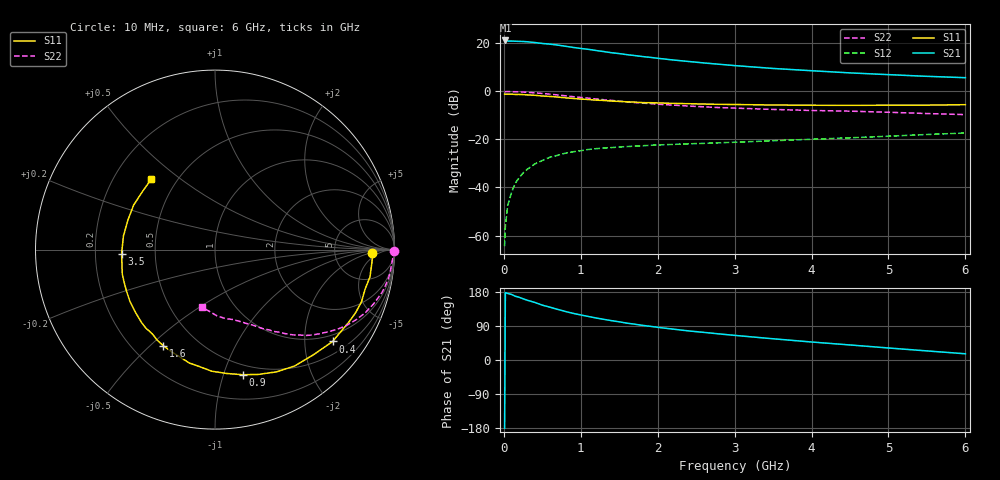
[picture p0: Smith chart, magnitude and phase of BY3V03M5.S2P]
! SIEMENS Small Signal Semiconductors
! BFY420
! Si NPN RF SIEGET Grounded Emitter Transistor in MICRO-X
! VCE = 3 V  IC = 3.5 mA
! Common Emitter S-Parameters:  October  1996
# GHz  S  MA  R  50
!  f  S11  S21  S12  S22
! GHz  MAG  ANG  MAG  ANG  MAG  ANG  MAG  ANG
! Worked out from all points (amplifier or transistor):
!   36 points, 10 MHz to 6 GHz, reference 50 ohm
!   highest |S21| = 21.2 dB at 20 MHz (marker M1)
!   |S21| within 3 dB of that: start of sweep to 924.5 MHz
!   unconditionally stable (mu >= 1): 3.483 GHz to end of sweep
!   at 250 MHz: K = 0.09, MSG = 27.4 dB, |S12| = -33.9 dB
!   at 1.4 GHz: K = 0.42, MSG = 19.7 dB, |S12| = -23.4 dB
!   at 6 GHz: K = 1.18, MAG = 9.0 dB, |S12| = -17.3 dB
!   S11 on the Smith chart (normalised r, x): 10 MHz: 15, -2; 400 MHz: 0.81, -2.69; 900 MHz: 0.41, -1.16; 1.6 GHz: 0.32, -0.55; 3.5 GHz: 0.32, -0.02; 6 GHz: 0.36, +0.39
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0.01  0.8764 -1.1  11.45 -180.0  0.0006 74.6  0.995 -0.4
0.02  0.8788 -2.2  11.51 177.9  0.0016 88.3  0.9864 -0.9
0.05  0.877 -5.0  11.19 175.6  0.0042 81.2  0.9926 -2.4
0.1  0.8767 -10.0  11.17 173.0  0.0079 83.1  0.9873 -4.9
0.15  0.8647 -14.7  11.09 168.2  0.0124 79.7  0.9842 -7.3
0.2  0.8665 -19.6  11.01 165.5  0.016 79.0  0.9794 -9.6
0.3  0.8474 -28.7  10.81 158.0  0.0236 74.3  0.9607 -14.4
0.4  0.8315 -38.0  10.44 152.1  0.0307 69.6  0.9347 -18.8
0.5  0.8031 -46.7  9.969 144.8  0.0364 65.0  0.9074 -22.9
0.6  0.7856 -55.6  9.645 139.3  0.0428 61.0  0.8765 -26.6
0.7  0.763 -63.2  9.223 133.6  0.0468 57.2  0.8441 -30.2
0.9  0.7137 -77.6  8.246 123.1  0.0554 51.0  0.7789 -36.0
1.1  0.6779 -91.5  7.512 114.8  0.0619 45.9  0.7221 -41.2
1.3  0.6479 -102.8  6.752 107.3  0.0665 42.0  0.6708 -45.2
1.6  0.6078 -118.3  5.825 97.2  0.0711 37.8  0.6049 -50.5
1.8  0.5849 -126.7  5.328 91.5  0.0738 35.4  0.5721 -53.2
2.2  0.5641 -141.9  4.511 81.5  0.0789 32.3  0.519 -58.4
2.8  0.5384 -160.0  3.677 68.8  0.0852 30.1  0.4605 -64.7
3.5  0.5208 -177.5  3.008 56.0  0.0941 28.6  0.4216 -71.3
4.5  0.5124 161.3  2.431 39.7  0.1082 26.0  0.3881 -81.6
5.5  0.518 140.8  2.061 24.0  0.1268 22.7  0.3461 -95.0
6  0.5292 132.1  1.932 16.4  0.1361 20.2  0.3291 -103.0
